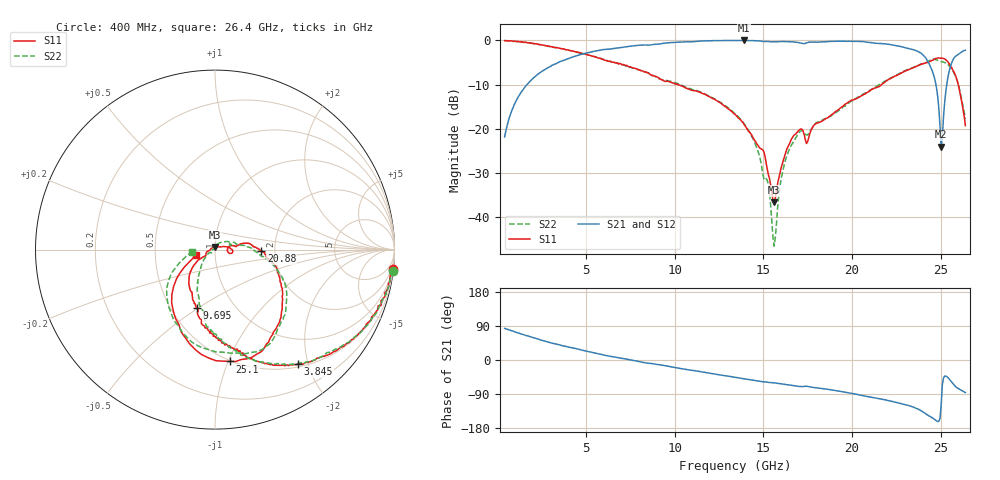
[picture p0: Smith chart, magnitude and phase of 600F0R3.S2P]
!  American Technical Ceramics  Date:  11/23/05
!  One Norden Lane
!  Huntington Station,  NY.  11746-2102
!  Tel:  (631) 622-4700  Fax:  (631) 622-4748
!  Part Number  600F0R3  Mounting Orientation: Horizontal
!  Description: Ultra Low ESR Microwave capacitors
!  Application: Coupling, Bypass, Tuning, DC Block
!  Filters, Matching
# GHZ S DB R 50
! Freq  |S11|  S11 Ph  |S21|  S21 Ph  |S12|  S12 Ph  |S22|  S22 Ph
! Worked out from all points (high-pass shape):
!   401 points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, 400 MHz to 26.4 GHz, reference 50 ohm
!   highest |S21| = 0.00 dB at 13.92 GHz (marker M1); lowest = -24.1 dB at 25.04 GHz (marker M2)
!   |S21| within 3 dB of the highest: 4.867 GHz to 23.94 GHz (19.07 GHz wide, 132 % of centre); 26.05 GHz to end of sweep
!   lowest |S11| = -36.7 dB at 15.61 GHz (marker M3), VSWR 1.03, Z = 49.9 + j1.46 ohm
!   |S11| at or under -10 dB: 10.19 GHz to 21.67 GHz (11.48 GHz wide, 72.1 % of centre); 26 GHz to end of sweep
!   |S22| runs from -46.5 to 0.0 dB; largest |S21 - S12| = 0.012
!   S11 on the Smith chart (normalised r, x): 400 MHz: 1, -18; 3.845 GHz: 0.55, -1.83; 9.695 GHz: 0.67, -0.49; 20.88 GHz: 1.70, -0.02; 25.1 GHz: 0.49, -1.01; 26.4 GHz: 0.81, -0.05
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0.4  -0.04 -6.2  -21.85 83.4  -21.86 83.3  -0.03 -6.8
1.57  -0.40 -24.3  -10.42 65.0  -10.44 65.4  -0.42 -25.0
3.845  -2.08 -54.0  -4.34 35.8  -4.39 35.6  -2.09 -53.6
4.755  -2.92 -63.5  -3.12 26.4  -3.15 26.2  -2.93 -62.7
9.11  -8.50 -104.7  -0.81 -12.3  -0.82 -12.1  -8.68 -99.5
9.695  -9.32 -107.3  -0.52 -17.2  -0.52 -17.1  -9.19 -101.3
13.4  -16.76 -143.8  -0.01 -45.8  -0.01 -45.8  -16.59 -125.0
13.92  -19.07 -148.1  0.00 -49.8  -0.01 -49.6  -18.86 -131.2
15.22  -29.14 -170.3  -0.22 -58.6  -0.20 -58.6  -31.67 -144.2
15.61  -36.66 93.6  -0.29 -60.3  -0.26 -60.3  -46.55 145.9
16  -28.87 24.8  -0.24 -62.9  -0.22 -63.0  -31.28 72.5
16.39  -24.00 14.8  -0.28 -65.5  -0.25 -65.5  -25.38 49.6
17.755  -19.79 12.2  -0.36 -72.0  -0.38 -72.4  -19.81 22.9
20.875  -11.73 -1.4  -0.38 -96.5  -0.37 -96.3  -11.68 -8.0
22.11  -8.70 -18.5  -0.90 -107.8  -0.91 -107.5  -8.68 -18.7
24.19  -5.05 -53.3  -4.12 -142.8  -4.12 -142.5  -5.00 -51.5
24.645  -4.23 -63.6  -8.33 -156.2  -8.35 -155.9  -4.24 -68.0
25.035  -3.96 -79.5  -24.05 -117.8  -23.68 -117.4  -4.78 -83.9
25.1  -4.03 -82.4  -21.93 -65.5  -21.74 -66.5  -4.85 -86.4
25.555  -5.76 -109.0  -5.93 -54.2  -5.93 -54.3  -6.10 -111.7
25.945  -9.20 -133.9  -3.29 -73.8  -3.27 -74.0  -9.20 -141.2
26.4  -19.29 -163.2  -2.22 -86.0  -2.21 -85.8  -17.77 -175.1
